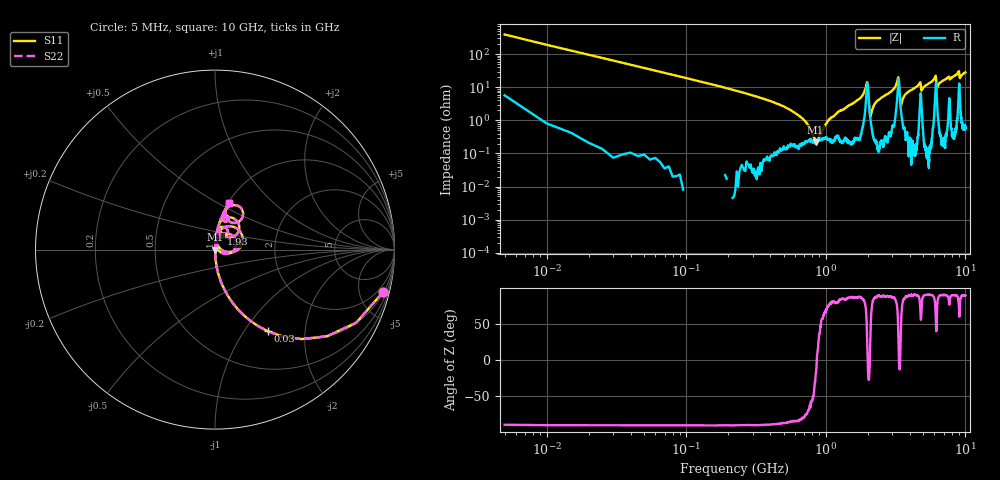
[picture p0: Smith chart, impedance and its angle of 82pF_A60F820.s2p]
! Amotech Co.,Ltd.
! http://www.amotech.co.kr/
! Part Number: A60F820
! These Parameters are Measured in Series Mode Connection
! Operation Temp=25[degC], DC Bias Voltage=0[V]
! Freq. Start=5[MHz] Stop=10[GHz], 2000[Steps]
! Date: Monday, July 20, 2020, 03:43:59
# GHZ S RI R 50.000000
!Freq.(Hz) S11(Real) S11(Imag) S21(Real) S21(Imag) S12(Real) S12(Imag) S22(Real) S22(Imag)
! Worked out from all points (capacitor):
!   2000 points, 5 MHz to 10 GHz, reference 50 ohm
!   read as one part in series: C = 82.5 pF near 55 MHz
!   lowest |Z| = 216 mohm at 845 MHz (marker M1)
!   series resonance near 862.1 MHz, so ESL is about 410 pH
!   S11 on the Smith chart (normalised r, x): 5 MHz: 1.11, -7.92; 30 MHz: 1.00, -1.29; 1.93 GHz: 1.06, +0.18; 10 GHz: 1.01, +0.57
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0.005  0.937 -0.2358  0.063 0.2358  0.063 0.2358  0.937 -0.2358
0.03  0.2931 -0.4546  0.7069 0.4546  0.7069 0.4546  0.2931 -0.4546
0.125  0.0223 -0.148  0.9777 0.148  0.9777 0.148  0.0223 -0.148
0.67  0.00185 -0.0119  0.9981 0.0119  0.9981 0.0119  0.00185 -0.0119
0.845  0.00201 -0.000779  0.998 0.000779  0.998 0.000779  0.00201 -0.000779
1.09  0.00277 0.0115  0.9972 -0.0115  0.9972 -0.0115  0.00277 0.0115
1.675  0.00448 0.0399  0.9955 -0.0399  0.9955 -0.0399  0.00448 0.0399
1.93  0.0358 0.0849  0.9642 -0.0849  0.9642 -0.0849  0.0358 0.0849
1.985  0.1185 0.0267  0.8815 -0.0267  0.8815 -0.0267  0.1185 0.0267
2.105  0.00833 0.0117  0.9917 -0.0117  0.9917 -0.0117  0.00833 0.0117
2.35  0.00312 0.0397  0.9969 -0.0397  0.9969 -0.0397  0.00312 0.0397
3.28  0.1037 0.1263  0.8963 -0.1263  0.8963 -0.1263  0.1037 0.1263
3.34  0.1329 0.00389  0.8671 -0.00389  0.8671 -0.00389  0.1329 0.00389
3.46  0.018 0.0202  0.982 -0.0202  0.982 -0.0202  0.018 0.0202
3.885  0.00751 0.0717  0.9925 -0.0717  0.9925 -0.0717  0.00751 0.0717
4.715  0.0404 0.1271  0.9596 -0.1271  0.9596 -0.1271  0.0404 0.1271
5.005  0.0133 0.0983  0.9867 -0.0983  0.9867 -0.0983  0.0133 0.0983
6.085  0.091 0.1782  0.909 -0.1782  0.909 -0.1782  0.091 0.1782
6.26  0.042 0.0794  0.958 -0.0794  0.958 -0.0794  0.042 0.0794
6.67  0.0237 0.1409  0.9763 -0.1409  0.9763 -0.1409  0.0237 0.1409
8.335  0.0509 0.2113  0.9491 -0.2113  0.9491 -0.2113  0.0509 0.2113
10  0.0793 0.2592  0.9207 -0.2592  0.9207 -0.2592  0.0793 0.2592
